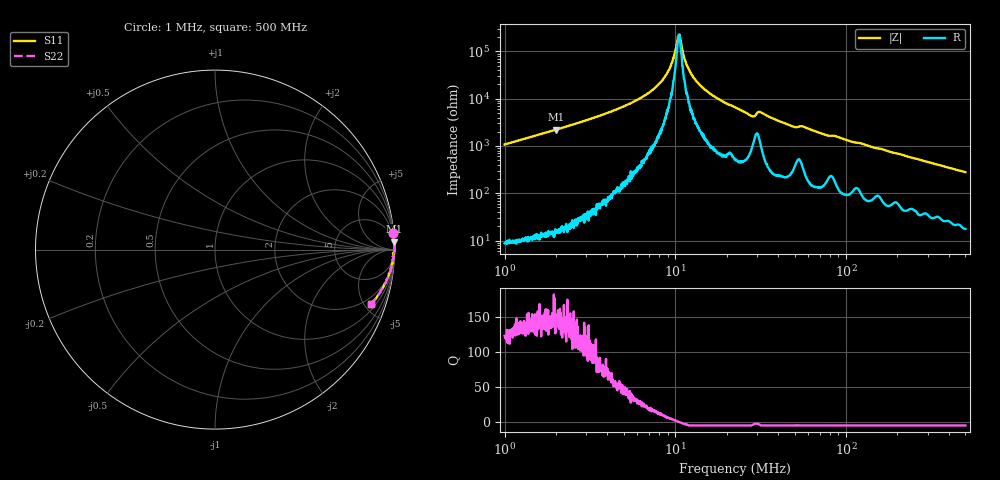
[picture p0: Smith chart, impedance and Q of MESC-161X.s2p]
!s-Parameter Generated by FASTRON Sdn. Bhd.
!FASTRON P/N : MESC-161X
!Keysight Technologies,E4991B,MY54100416,A.01.15
!Date: Fri Mar 27 10:48:43 2026
!Version  : Rev00 Fri Mar 27 10:48:43 2026
!Data & Calibration Information:
!PortZ  Port1:50+j0  Port2:50+j0
!When reading, reference impedance value at option line is always used.
! Remarks : This data is being provided solely for informational purposes.
!Freq	S11	S21	S12	S22
# Hz S dB R 50
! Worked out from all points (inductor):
!   1601 points, 1 MHz to 500 MHz, reference 50 ohm
!   read as one part in series: L = 170 uH near 1.032 MHz
!   highest Q = 155 at 1.996 MHz (marker M1), where L = 176 uH
!   self-resonance near 10.48 MHz
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1000000  -0.04 5.3  -20.69 -84.2  -20.69 -84.2  -0.04 5.3
1996459  -0.01 2.6  -26.90 -87.0  -26.90 -87.0  -0.01 2.6
2820919  -0.01 1.8  -30.25 -87.7  -30.25 -87.7  -0.01 1.8
5566606  -0.00 0.7  -38.31 -87.7  -38.31 -87.7  -0.00 0.7
7957584  -0.00 0.3  -46.01 -85.5  -46.01 -85.5  -0.00 0.3
9295130  -0.00 0.1  -53.03 -78.4  -53.03 -78.4  -0.00 0.1
9814575  -0.00 0.1  -57.97 -70.7  -57.97 -70.7  -0.00 0.1
1.028286e7  -0.00 0.0  -64.67 -43.1  -64.67 -43.1  -0.00 0.0
1.052531e7  -0.00 -0.0  -66.39 6.4  -66.39 6.4  -0.00 -0.0
1.073172e7  -0.00 -0.0  -64.78 39.5  -64.78 39.5  -0.00 -0.0
1.128751e7  -0.00 -0.1  -57.17 69.8  -57.17 69.8  -0.00 -0.1
1.168907e7  -0.00 -0.1  -54.10 74.5  -54.10 74.5  -0.00 -0.1
1.328759e7  -0.00 -0.2  -47.45 82.7  -47.45 82.7  -0.00 -0.2
1.63884e7  -0.01 -0.5  -41.63 85.0  -41.63 85.0  -0.01 -0.5
2.236068e7  -0.01 -0.9  -36.41 84.5  -36.41 84.5  -0.01 -0.9
2.801062e7  -0.04 -1.3  -32.69 76.7  -32.69 76.7  -0.04 -1.3
3.147229e7  -0.04 -1.1  -34.38 76.3  -34.38 76.3  -0.04 -1.1
4.843613e7  -0.04 -2.2  -28.37 81.5  -28.37 81.5  -0.04 -2.2
5.548932e7  -0.05 -2.2  -28.36 79.7  -28.36 79.7  -0.05 -2.2
6.307767e7  -0.04 -2.6  -26.78 83.6  -26.78 83.6  -0.04 -2.6
1.77937e8  -0.15 -7.3  -17.86 78.6  -17.86 78.6  -0.15 -7.3
5e8  -0.70 -19.3  -9.60 67.1  -9.60 67.1  -0.70 -19.3
